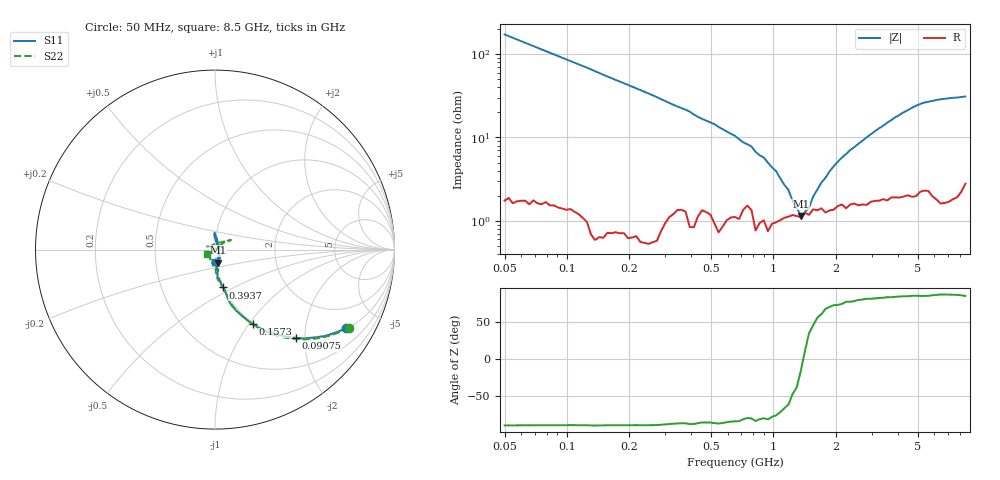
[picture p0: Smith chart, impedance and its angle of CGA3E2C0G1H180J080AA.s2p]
! S-parameter Generated by TDK Corporation
! Copyright(C) 2015 TDK Corporation.
! All Rights Reserved.
! TDK P/N: CGA3E2C0G1H180J080AA (Multilayer Ceramic Chip Capacitors)
! Property: C=18pF
! Size(LxWxT): 1.6x0.8x0.8mm, 0.063x0.031x0.031inches
! Model Type: s2p (Touchstone File Format Version 1.0)
! Frequency: DC=Yes Start=50MHz Stop=8500MHz 114points Log-sweep
! Note:
! Model Generated on Jun. 23, 2015
! Hash(MD5):
! Port Assignments:
!  1 ---| |--- 2
! Applicable Conditions:
!  Temperature = 25 degC
!  DC Bias Voltage = 0 V
!  Small Signal Operation
! Terms and conditions regarding TDK Simulation Models
! (1)This simulation model is being provided solely for informational purposes. Please refer to the specifications of the products in terms of detailed characteristics of such products.
! (2)In no event shall TDK Corporation of any of its subsidiaries be liable for any loss or damage arising, directly or indirectly,
!  From any information contained in this simulation model, including, but not limited to loss or damages arising from any inaccuracies, omissions or errors in connection with such information.
! (3)Any and all copyrights on this simulation model are owned by TDK Corporation.
!  Duplication or redistribution of this simulation model without prior written permission from TDK Corporation is prohibited.
! (4)This simulation model is subject to any modification or change without any prior notice.
! (5)Neither TDK Corporation nor any of its subsidiaries shall make any warranty, express or implied,
!  Including but not limited to the correctness, implied warranties of merchantability and fitness for a particular purpose with respect to this simulation models.
! (6)The use of this simulation model shall be deemed to have consented to the terms and conditions hereof.
# MHz S MA R 50
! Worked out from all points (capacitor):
!   113 points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, 50 MHz to 8.5 GHz, reference 50 ohm
!   read as one part in series: C = 18.5 pF near 50 MHz
!   lowest |Z| = 1.15 ohm at 1.358 GHz (marker M1)
!   series resonance near 1.394 GHz, so ESL is about 700 pH
!   S11 on the Smith chart (normalised r, x): 50 MHz: 1.05, -3.33; 90.75 MHz: 1.02, -1.82; 157.3 MHz: 0.98, -1.05; 393.7 MHz: 0.99, -0.44; 8.5 GHz: 0.99, -0.14
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50  0.8512 -30.8  0.4984 59.0  0.499 59.0  0.8634 -30.2
90.75308  0.6687 -47.4  0.7127 42.6  0.7123 42.6  0.6893 -46.5
119.495  0.5689 -54.9  0.7951 35.0  0.7952 35.0  0.5884 -54.5
157.3396  0.4674 -63.0  0.8647 27.6  0.8637 27.7  0.4813 -61.9
285.5811  0.2911 -74.9  0.9415 15.1  0.9426 15.2  0.2814 -75.3
393.6702  0.2154 -78.5  0.9628 10.2  0.9639 10.3  0.2151 -79.1
651.9202  0.1353 -84.1  0.969 4.0  0.9701 4.1  0.1299 -87.6
1357.782  0.07393 -76.6  0.9772 -3.5  0.9785 -3.6  0.06481 -109.1
1558.024  0.06601 -71.9  0.9737 -5.1  0.9743 -5.1  0.06059 -113.9
2147.718  0.0526 -57.8  0.9738 -8.7  0.9721 -8.7  0.04573 -129.8
2827.91  0.029 -36.4  0.9721 -12.5  0.9731 -12.4  0.02805 -142.1
3099.524  0.02259 -7.2  0.9706 -13.9  0.9694 -13.8  0.01556 -153.3
3244.963  0.01699 10.1  0.9693 -14.6  0.9694 -14.6  0.006469 -173.9
3397.226  0.02119 30.1  0.9708 -15.4  0.9692 -15.4  0.002281 103.3
3556.634  0.02553 62.6  0.9694 -16.2  0.9687 -16.2  0.01409 53.2
3723.522  0.03098 69.0  0.9685 -17.1  0.9673 -17.1  0.02405 42.3
4272.658  0.06324 88.9  0.9627 -19.8  0.9651 -19.9  0.06169 38.5
5132.831  0.09217 91.9  0.9572 -24.3  0.9555 -24.3  0.1022 32.5
6166.175  0.0746 86.0  0.9572 -29.2  0.9579 -29.0  0.08139 35.7
7075.547  0.02559 36.1  0.9586 -33.9  0.9571 -33.7  0.03892 71.0
7407.553  0.0259 -23.6  0.9563 -35.6  0.9592 -35.6  0.02944 103.4
8500  0.07033 -90.5  0.9445 -42.0  0.9446 -41.9  0.04964 -151.7
